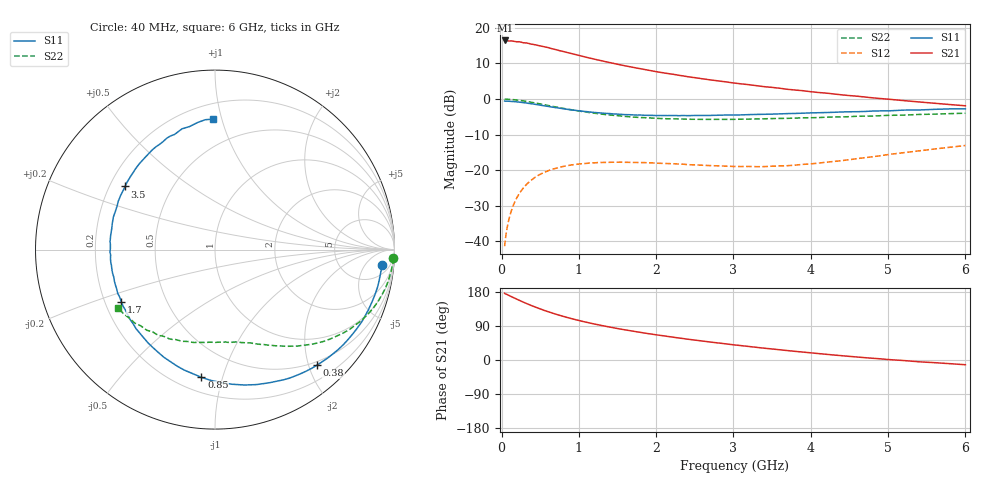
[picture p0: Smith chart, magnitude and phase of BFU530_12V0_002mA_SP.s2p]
! Filename:  P:\Prog\Test\Noise\ATS_data\Testdata_Net\03 Spar\BFU530_APG2013_40_A05_12p0V_002mA_SP_CM01_D.s2p
! Date/Time: Fri 26/Apr/2013 13:03:12
! BFU530_APG2013_40_A05_12p0V_1to25mA_SP_CM01_Bias2_R.s2p
! MDIF S-parameter v. bias file
! BFU530_APG2013_40_A05_12p0V_1to25mA_SP_CM01
! Date/time Wed Apr 24 20:41:12 2013
! VAR V_out= 12.0000
! VAR I_out= 2.0000
! VAR V_in= 0.7918
! VAR I_in= 0.0174
! Device data file deembeded for feedlines and parallel
! Original file: \03 Spar\BFU530_APG2013_40_A05_12p0V_002mA_SP_CM01_R.s2p
! Feed-files: PR047V01_250413_Feed1.s2p, PR047V01_250413_Feed2.s2p
! Parallel-file: PR047V01_250413_Par.s2p
# MHz S MA R 50
!  Freq-MHz  S11-mag  S11-arg  S21-mag  S21-arg  S12-mag  S12-arg  S22-mag  S22-arg
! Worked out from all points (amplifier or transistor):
!   98 points, 40 MHz to 6 GHz, reference 50 ohm
!   highest |S21| = 16.5 dB at 50 MHz (marker M1)
!   |S21| within 3 dB of that: start of sweep to 776.9 MHz
!   unconditionally stable (mu >= 1): 2.906 GHz to 4.76 GHz
!   at 300 MHz: K = 0.11, MSG = 20.2 dB, |S12| = -24.6 dB
!   at 1.6 GHz: K = 0.54, MSG = 13.6 dB, |S12| = -17.8 dB
!   at 6 GHz: K = 0.80, MSG = 5.6 dB, |S12| = -13.1 dB
!   S11 on the Smith chart (normalised r, x): 40 MHz: 10, -14; 380 MHz: 0.44, -2.14; 850 MHz: 0.29, -0.86; 1.7 GHz: 0.27, -0.24; 3.5 GHz: 0.26, +0.30; 6 GHz: 0.30, +0.94
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40  0.9355 -5.3  6.657 176.1  0.008484 85.5  0.9949 -2.8
50  0.9336 -6.6  6.664 174.4  0.01062 84.9  0.9955 -3.6
70  0.9312 -9.1  6.606 173.1  0.01487 83.6  0.9919 -5.2
120  0.9257 -15.9  6.584 167.9  0.02523 79.8  0.9842 -8.8
240  0.8997 -31.5  6.353 156.5  0.0485 70.6  0.954 -17.4
320  0.8773 -41.4  6.15 149.4  0.06216 64.8  0.9256 -22.8
380  0.8588 -48.5  5.927 144.2  0.0713 60.7  0.9012 -26.5
460  0.8334 -57.8  5.716 137.9  0.08235 55.8  0.8703 -30.9
600  0.7869 -72.9  5.298 127.7  0.09747 48.0  0.8114 -38.0
700  0.7563 -82.7  4.964 121.0  0.1056 43.2  0.7731 -42.3
850  0.7158 -96.1  4.508 112.2  0.1152 37.1  0.7215 -47.7
1050  0.6713 -111.9  3.982 101.8  0.1229 30.5  0.6642 -54.2
1200  0.6459 -122.5  3.64 95.0  0.1264 26.5  0.6306 -58.1
1350  0.6266 -131.8  3.343 88.9  0.1282 23.2  0.6029 -61.7
1700  0.5975 -150.8  2.791 76.2  0.1279 17.7  0.5564 -69.1
2050  0.5855 -166.8  2.374 65.1  0.1243 14.5  0.5313 -75.9
2500  0.5863 175.8  1.996 52.6  0.1182 13.7  0.518 -84.2
3100  0.5973 155.8  1.632 37.9  0.112 18.2  0.5195 -95.2
3500  0.6125 144.9  1.456 29.1  0.1133 23.6  0.5303 -102.5
4100  0.6409 129.1  1.234 17.0  0.1251 31.6  0.5474 -113.8
5200  0.6976 105.3  0.9491 -1.4  0.1755 37.0  0.5927 -134.2
6000  0.727 90.8  0.8023 -12.5  0.2215 33.5  0.6305 -148.8
